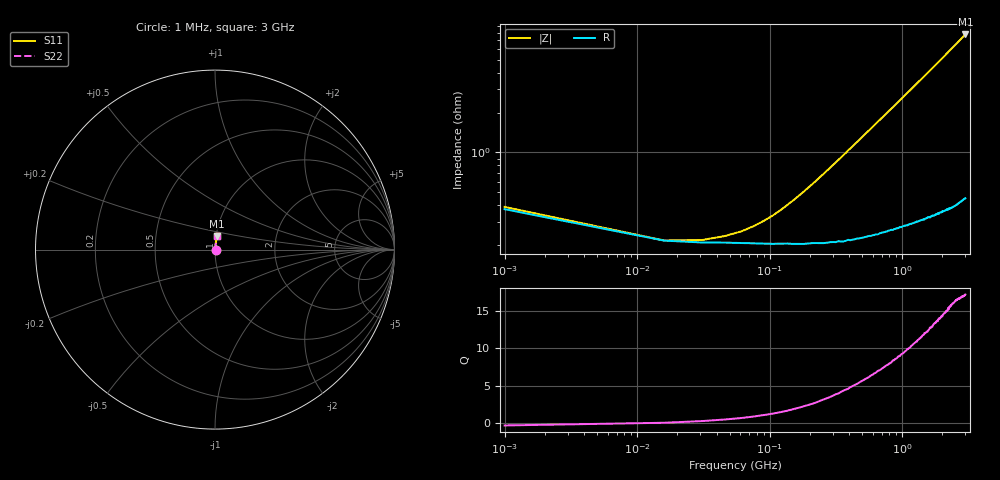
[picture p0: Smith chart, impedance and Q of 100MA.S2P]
!Keysight Technologies,E4991B,MY54301043,A.02.04
!Date: Thu Nov 16 21:15:49 2023
!Data:
!Freq	S11	S21	S12	S22
# Hz S MA R 50
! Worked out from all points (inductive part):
!   201 points, 1 MHz to 3 GHz, reference 50 ohm
!   read as one part in series: L = 411 pH near 240.9 MHz
!   highest Q = 17.2 at 3 GHz (marker M1), where L = 411 pH
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1000000  0.00387 -15.9  0.9963 0.1  0.9963 0.1  0.00387 -15.9
1.5995e7  0.002165 4.2  0.9978 -0.0  0.9978 -0.0  0.002165 4.2
3.099e7  0.002182 16.6  0.9979 -0.0  0.9979 -0.0  0.002182 16.6
6.098e7  0.002532 35.0  0.9979 -0.1  0.9979 -0.1  0.002532 35.0
1.2096e8  0.003669 55.9  0.998 -0.2  0.998 -0.2  0.003669 55.9
1.5095e8  0.004348 61.8  0.998 -0.2  0.998 -0.2  0.004348 61.8
1.95935e8  0.005426 67.5  0.9979 -0.3  0.9979 -0.3  0.005426 67.5
2.4092e8  0.006545 71.3  0.9979 -0.4  0.9979 -0.4  0.006545 71.3
3.009e8  0.008043 74.4  0.9979 -0.4  0.9979 -0.4  0.008043 74.4
3.6088e8  0.00954 76.6  0.9978 -0.5  0.9978 -0.5  0.00954 76.6
4.35855e8  0.01146 78.3  0.9977 -0.6  0.9977 -0.6  0.01146 78.3
5.1083e8  0.01336 79.4  0.9976 -0.8  0.9976 -0.8  0.01336 79.4
6.008e8  0.01562 80.4  0.9975 -0.9  0.9975 -0.9  0.01562 80.4
7.05765e8  0.01826 81.2  0.9974 -1.0  0.9974 -1.0  0.01826 81.2
8.25725e8  0.02128 81.8  0.9972 -1.2  0.9972 -1.2  0.02128 81.8
1.005665e9  0.02578 82.4  0.9969 -1.5  0.9969 -1.5  0.02578 82.4
1.26058e9  0.03219 82.9  0.9965 -1.8  0.9965 -1.8  0.03219 82.9
1.5005e9  0.03824 83.1  0.9961 -2.2  0.9961 -2.2  0.03824 83.1
1.725425e9  0.04397 83.2  0.9957 -2.5  0.9957 -2.5  0.04397 83.2
2.01033e9  0.05125 83.1  0.9951 -2.9  0.9951 -2.9  0.05125 83.1
2.505165e9  0.06413 82.8  0.994 -3.7  0.994 -3.7  0.06413 82.8
3e9  0.07702 82.3  0.9926 -4.4  0.9926 -4.4  0.07702 82.3
